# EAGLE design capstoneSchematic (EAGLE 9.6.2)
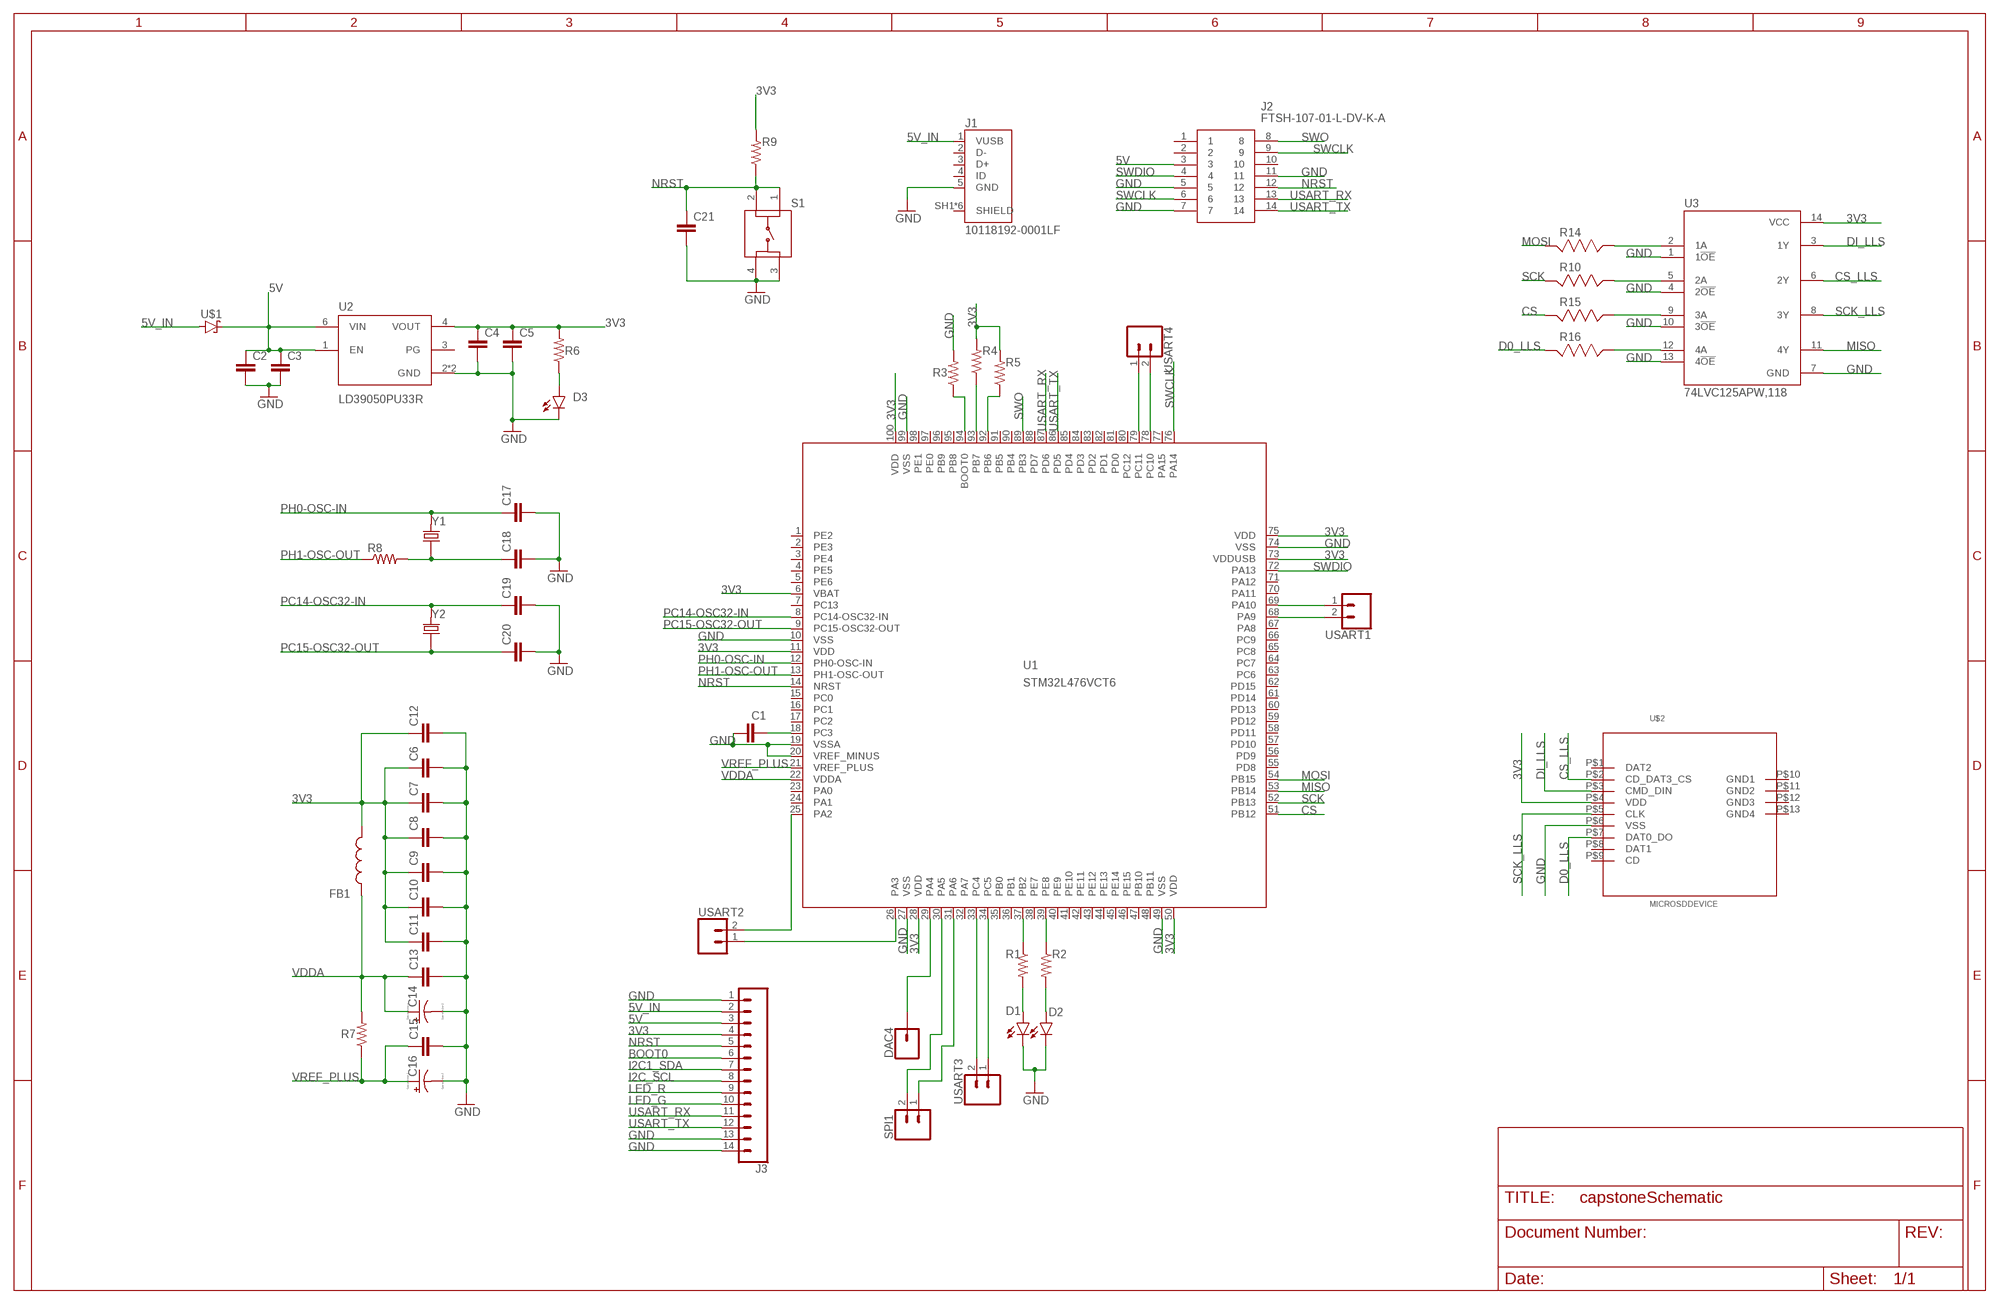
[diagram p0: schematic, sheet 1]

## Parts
C1  CC0603KRX5R7BB105  [CAPC1608X90]
C2  CC0603KRX5R7BB105  [CAPC1608X90]
C3  CC0402KRX7R7BB104  [CAPC1005X55N]
C4  CC0603KRX5R7BB105  [CAPC1608X90]
C5  CC0402KRX7R7BB104  [CAPC1005X55N]
C6  CC0402KRX7R7BB104  [CAPC1005X55N]
C7  CC0402KRX7R7BB104  [CAPC1005X55N]
C8  CC0402KRX7R7BB104  [CAPC1005X55N]
C9  CC0402KRX7R7BB104  [CAPC1005X55N]
C10  CC0402KRX7R7BB104  [CAPC1005X55N]
C11  CC0402KRX7R7BB104  [CAPC1005X55N]
C12  CC0603KRX5R7BB105  [CAPC1608X90]
C13  CC0402KRX7R7BB104  [CAPC1005X55N]
C14  TAJA105K016RNJ  [CAPPM3216X180N]
C15  CC0402KRX7R7BB104  [CAPC1005X55N]
C16  TAJA105K016RNJ  [CAPPM3216X180N]
C17  CC0402JRNPO9BN200  [CAPC1005X55N]
C18  CC0402JRNPO9BN200  [CAPC1005X55N]
C19  CC0402CRNPO9BN4R7  [CAPC1005X55N]
C20  CC0402CRNPO9BN4R7  [CAPC1005X55N]
C21  CC0402KRX7R7BB104  [CAPC1005X55N]
D1  SML-P12MTT86  [LED_SML-P11UTT86R]
D2  SML-P12MTT86  [LED_SML-P11UTT86R]
D3  SML-P12MTT86  [LED_SML-P11UTT86R]
DAC4  CONN_01  [1X01]
FB1  BK1608HS601-T  [BEADC1608X95N]
J1  10118192-0001LF  [AMPHENOL_10118192-0001LF]
J2  FTSH-107-01-L-DV-K-A  [FTSH10701LDVKA]
J3  CONN_14  [1X14]
R1  RC0402FR-071KL  [RESC1005X40N]
R2  RC0402FR-071KL  [RESC1005X40N]
R3  RC0402FR-071KL  [RESC1005X40N]
R4  RC0402FR-071KL  [RESC1005X40N]
R5  RC0402FR-071KL  [RESC1005X40N]
R6  RC0402FR-071KL  [RESC1005X40N]
R7  RC0402FR-071KL  [RESC1005X40N]
R8  RC0402FR-072KL  [RESC1005X40N]
R9  RC0402FR-0710KL  [RESC1005X40N]
R10  RC0402FR-073K3L  [RESC1005X40]
R14  RC0402FR-073K3L  [RESC1005X40]
R15  RC0402FR-073K3L  [RESC1005X40]
R16  RC0402FR-073K3L  [RESC1005X40]
S1  LL3301FF065QJ  [LL3301FF065QJ]
SPI1  CONN_02  [1X02]
U1  STM32L476VCT6  [LQFP100_14X14]
U2  LD39050PU33R  [SON95P300X300X100-7N]
U3  74LVC125APW,118  [IC_74LVC125APW,118]
U$1  STPS1L30A  [DIOM5226X223N]
U$2  MICROSDDEVICE  [MICROSD]
USART1  CONN_02  [1X02]
USART2  CONN_02  [1X02]
USART3  CONN_02  [1X02]
USART4  CONN_02  [1X02]
Y1  ABLS-8.000MHZ-B2-T  [XTAL_ABLS-8.000MHZ-B2-T]
Y2  ECS-.327-12.5-12QS-TR  [XTAL_ECS-.327-12.5-12QS-TR]

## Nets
3V3: C4.1 C5.1 C6.1 C7.1 C8.1 C9.1 C10.1 C11.1 C12.1 FB1.2 J3.4 R4.2 R5.2 R6.2 R9.2 U1.6(VBAT) U1.11(VDD) U1.28(VDD) U1.50(VDD) U1.73(VDDUSB) U1.75(VDD) U1.100(VDD) U2.4(VOUT) U3.14(VCC) U$2.P$4(VDD)
5V: C2.1 C3.1 J2.3 J3.3 U2.1(EN) U2.6(VIN) U$1.1(C)
5V_IN: J1.1(VUSB) J3.2 U$1.2(A)
BOOT0: J3.6
CS: R15.1 U1.51(PB12)
CS_LLS: U3.6(2Y) U$2.P$2(CD_DAT3_CS)
D0_LLS: R16.1 U$2.P$7(DAT0_DO)
DI_LLS: U3.3(1Y) U$2.P$3(CMD_DIN)
GND: C1.1 C2.2 C3.2 C4.2 C5.2 C6.2 C7.2 C8.2 C9.2 C10.2 C11.2 C12.2 C13.2 C14.C(-) C15.2 C16.C(-) C17.2 C18.2 C19.2 C20.2 C21.2 D1.C D2.C D3.C J1.5(GND) J2.5 J2.7 J2.11 J3.1 J3.13 J3.14 R3.2 S1.3 S1.4 U1.10(VSS) U1.19(VSSA) U1.20(VREF_MINUS) U1.27(VSS) U1.49(VSS) U1.74(VSS) U1.99(VSS) U2.2(GND) U2.7(GND) U3.1(1!OE) U3.4(2!OE) U3.7(GND) U3.10(3!OE) U3.13(4!OE) U$2.P$6(VSS)
I2C1_SDA: J3.7
I2C_SCL: J3.8
LED_G: J3.10
LED_R: J3.9
MISO: U1.53(PB14) U3.11(4Y)
MOSI: R14.1 U1.54(PB15)
N$1: R2.1 U1.39(PE8)
N$2: R1.1 U1.37(PB2)
N$3: D1.A R1.2
N$4: D2.A R2.2
N$5: R3.1 U1.94(BOOT0)
N$6: R4.1 U1.93(PB7)
N$7: R5.1 U1.92(PB6)
N$8: D3.A R6.1
N$9: U1.33(PC4) USART3.2
N$10: C1.2 U1.18(PC3)
N$11: U1.34(PC5) USART3.1
N$12: C18.1 R8.2 Y1.1
N$13: R14.2 U3.2(1A)
N$14: U1.78(PC10) USART4.2
N$15: DAC4.1 U1.29(PA4)
N$16: U1.79(PC11) USART4.1
N$17: SPI1.2 U1.30(PA5)
N$18: SPI1.1 U1.31(PA6)
N$19: U1.69(PA10) USART1.1
N$20: U1.68(PA9) USART1.2
N$22: U1.25(PA2) USART2.2
N$23: U1.26(PA3) USART2.1
N$24: R10.2 U3.5(2A)
N$25: R15.2 U3.9(3A)
N$26: R16.2 U3.12(4A)
NRST: C21.1 J2.12 J3.5 R9.1 S1.1 S1.2 U1.14(NRST)
PC14-OSC32-IN: C19.1 U1.8(PC14-OSC32-IN) Y2.2
PC15-OSC32-OUT: C20.1 U1.9(PC15-OSC32-OUT) Y2.1
PH0-OSC-IN: C17.1 U1.12(PH0-OSC-IN) Y1.2
PH1-OSC-OUT: R8.1 U1.13(PH1-OSC-OUT)
SCK: R10.1 U1.52(PB13)
SCK_LLS: U3.8(3Y) U$2.P$5(CLK)
SWCLK: J2.6 J2.9 U1.76(PA14)
SWDIO: J2.4 U1.72(PA13)
SWO: J2.8 U1.89(PB3)
USART_RX: J2.13 J3.11 U1.87(PD6)
USART_TX: J2.14 J3.12 U1.86(PD5)
VDDA: C13.1 C14.A(+) FB1.1 R7.2 U1.22(VDDA)
VREF_PLUS: C15.1 C16.A(+) R7.1 U1.21(VREF_PLUS)
Unconnected: J1.2(D-) J1.3(D+) J1.4(ID) J1.SH1(SHIELD) J1.SH2(SHIELD) J1.SH3(SHIELD) J1.SH4(SHIELD) J1.SH5(SHIELD) J1.SH6(SHIELD) J2.1 J2.2 J2.10 U1.1(PE2) U1.2(PE3) U1.3(PE4) U1.4(PE5) U1.5(PE6) U1.7(PC13) U1.15(PC0) U1.16(PC1) U1.17(PC2) U1.23(PA0) U1.24(PA1) U1.32(PA7) U1.35(PB0) U1.36(PB1) U1.38(PE7) U1.40(PE9) U1.41(PE10) U1.42(PE11) U1.43(PE12) U1.44(PE13) U1.45(PE14) U1.46(PE15) U1.47(PB10) U1.48(PB11) U1.55(PD8) U1.56(PD9) U1.57(PD10) U1.58(PD11) U1.59(PD12) U1.60(PD13) U1.61(PD14) U1.62(PD15) U1.63(PC6) U1.64(PC7) U1.65(PC8) U1.66(PC9) U1.67(PA8) U1.70(PA11) U1.71(PA12) U1.77(PA15) U1.80(PC12) U1.81(PD0) U1.82(PD1) U1.83(PD2) U1.84(PD3) U1.85(PD4) U1.88(PD7) U1.90(PB4) U1.91(PB5) U1.95(PB8) U1.96(PB9) U1.97(PE0) U1.98(PE1) U2.3(PG) U$2.P$1(DAT2) U$2.P$8(DAT1) U$2.P$9(CD) U$2.P$10(GND1) U$2.P$11(GND2) U$2.P$12(GND3) U$2.P$13(GND4)

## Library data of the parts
C1 C2 C4 C12 = ce-capstone:CC0603KRX5R7BB105: CAPACITOR CERAMIC, 1µF, 10V, X5R, 0603; Dielectric Characteristic:X5R; Capacitance:1µF; Capacitance Tolerance:± 10%; Voltage Rating:16V; Temperature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; DESCRIPTION: 1µF ±10% 16V Ceramic Capacitor X5R 0603 _1608 Metric_; DIGI-KEY_PART_NUMBER: 311-1444-1-ND; DIGI-KEY_PURCHASE_URL: https://www.digikey.com/product-detail/en/yageo/CC0603KRX5R7BB105/311-1444-1-ND/2833750?utm_source=snapeda&utm_medium=aggregator&utm_campaign=symbol; MF: Yageo; MP: CC0603KRX5R7BB105; PACKAGE: 0603 Yageo
C3 C5-C11 C13 C15 C21 = ce-capstone:CC0402KRX7R7BB104: .1UF 16V 10% 0402; DESCRIPTION: 0.1µF ±10% 16V Ceramic Capacitor X7R 0402 _1005 Metric_; DIGI-KEY_PART_NUMBER: 311-1338-1-ND; DIGI-KEY_PURCHASE_URL: https://www.digikey.com/product-detail/en/yageo/CC0402KRX7R7BB104/311-1338-1-ND/2103122?utm_source=snapeda&utm_medium=aggregator&utm_campaign=symbol; MF: Yageo; MP: CC0402KRX7R7BB104; PACKAGE: 0402 Yageo
C14 C16 = ce-capstone:TAJA105K016RNJ: Capacitor tantalum TAJ 1206 1uF 16V AVX 1uF SMD Solid MnO2 Tantalum Electrolytic Capacitor, 16 V dc +/-10%, TAJ Series; ALLIED_NUMBER: 70474975; ALLIED_PRICE-STOCK: https://www.alliedelec.com/avx-taja105k016r/70474975/; DESCRIPTION: Capacitor tantalum TAJ 1206 1uF 16V AVX 1uF SMD Solid MnO2 Tantalum Electrolytic Capacitor, 16 V dc +/-10%, TAJ Series; HEIGHT: 1.8mm; MANUFACTURER_NAME: AVX; MANUFACTURER_PART_NUMBER: TAJA105K016RNJ; MOUSER_PART_NUMBER: 581-TAJA105K016RNJ; MOUSER_PRICE-STOCK: https://www.mouser.com/Search/Refine.aspx?Keyword=581-TAJA105K016R; RS_PART_NUMBER: 6992804P; RS_PRICE-STOCK: http://uk.rs-online.com/web/p/products/6992804P
C17 C18 = ce-capstone:CC0402JRNPO9BN200: CAPACITOR CERAMIC 20PF 50V, C0G, 0402; Dielectric Characteristic:C0G / NP0; Capacitance:20pF; Capacitance Tolerance:± 5%; Voltage Rating:50V; Capacitor Case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; DESCRIPTION: 20pF ±5% 50V Ceramic Capacitor C0G, NP0 0402 _1005 Metric_; DIGI-KEY_PART_NUMBER: 311-1417-1-ND; DIGI-KEY_PURCHASE_URL: https://www.digikey.com/product-detail/en/yageo/CC0402JRNPO9BN200/311-1417-1-ND/2833723?utm_source=snapeda&utm_medium=aggregator&utm_campaign=symbol; MF: Yageo; MP: CC0402JRNPO9BN200; PACKAGE: 0402 Yageo
C19 C20 = ce-capstone:CC0402CRNPO9BN4R7: 0402 4.7 pF 50 V ±0.25 pF Tolerance NP0 SMT Multilayer Ceramic Capacitor; DESCRIPTION: 4.7pF ±0.25pF 50V Ceramic Capacitor C0G, NP0 0402 _1005 Metric_; DIGI-KEY_PART_NUMBER: 311-1367-1-ND; DIGI-KEY_PURCHASE_URL: https://www.digikey.com/product-detail/en/yageo/CC0402CRNPO9BN4R7/311-1367-1-ND/2103151?utm_source=snapeda&utm_medium=aggregator&utm_campaign=symbol; MF: Yageo; MP: CC0402CRNPO9BN4R7; PACKAGE: 0402 Yageo
D1-D3 = ce-capstone:SML-P12MTT86: SML-P1 Series Red 0402 Clear 60 mcd 2 V Surface Mount PICOLED LED; AVAILABILITY: Unavailable; DESCRIPTION: Green 572nm LED Indication - Discrete 2V 0402 _1006 Metric_; MF: Rohm; MP: SML-P12MTT86; PACKAGE: 0402 Rohm; PRICE: None
DAC4 = SparkFun-Connectors:CONN_01: Single connection point. Often used as Generic Header-pin footprint for 0.1 inch spaced/style header connections
FB1 = ce-capstone:BK1608HS601-T: Ferrite Chip Bead(Lead Free); DESCRIPTION: Ferrite Chip Bead(Lead Free); HEIGHT: 0.95mm; MANUFACTURER_NAME: Taiyo Yuden; MANUFACTURER_PART_NUMBER: BK1608HS601-T
J1 = ce-capstone:10118192-0001LF: Single Port 5 Contact Horizontal Right Angle Shielded Micro B USB 2.0 Connector; AVAILABILITY: Unavailable; DESCRIPTION: USB - micro B USB 2.0 Receptacle Connector 5 Position Surface Mount, Right Angle; MF: Amphenol ICC; MP: 10118192-0001LF; PACKAGE: None; PRICE: None
J2 = ce-capstone:FTSH-107-01-L-DV-K-A: Headers & Wire Housings .050" Micro Terminal Strip Source: Datasheet; DESCRIPTION: Headers & Wire Housings .050" Micro Terminal Strip; HEIGHT: 5.97mm; MANUFACTURER_NAME: SAMTEC; MANUFACTURER_PART_NUMBER: FTSH-107-01-L-DV-K-A; MOUSER_PART_NUMBER: 200-FTSH10701LDVKA; MOUSER_PRICE-STOCK: https://www.mouser.com/Search/Refine.aspx?Keyword=200-FTSH10701LDVKA
J3 = SparkFun-Connectors:CONN_14: Multi connection point. Often used as Generic Header-pin footprint for 0.1 inch spaced/style header connections On any of the 0.1 inch spaced packages, you can populate with these: Break Away Headers - Straight (PRT-00116) Break Away Male Headers - Right Angle (PRT-00553) Female Headers (PRT-00115)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
R1-R7 = ce-capstone:RC0402FR-071KL: RES SMD 1k OHM 1% 1/16W 0402; DESCRIPTION: 510 Ohms ±1% 0.063W, 1/16W Chip Resistor 0402 _1005 Metric_ Moisture Resistant Thick Film; DIGI-KEY_PART_NUMBER: 311-510LRCT-ND; DIGI-KEY_PURCHASE_URL: https://www.digikey.com/product-detail/en/yageo/RC0402FR-07510RL/311-510LRCT-ND/729579?utm_source=snapeda&utm_medium=aggregator&utm_campaign=symbol; MF: Yageo; MP: RC0402FR-07510RL; PACKAGE: 1005 Panasonic Electronic Components
R8 = ce-capstone:RC0402FR-072KL: RES SMD 2k OHM 1% 1/16W 0402; DESCRIPTION: 510 Ohms ±1% 0.063W, 1/16W Chip Resistor 0402 _1005 Metric_ Moisture Resistant Thick Film; DIGI-KEY_PART_NUMBER: 311-510LRCT-ND; DIGI-KEY_PURCHASE_URL: https://www.digikey.com/product-detail/en/yageo/RC0402FR-07510RL/311-510LRCT-ND/729579?utm_source=snapeda&utm_medium=aggregator&utm_campaign=symbol; MF: Yageo; MP: RC0402FR-07510RL; PACKAGE: 1005 Panasonic Electronic Components
R9 = ce-capstone:RC0402FR-0710KL: RES SMD 10k OHM 1% 1/16W 0402; DESCRIPTION: 510 Ohms ±1% 0.063W, 1/16W Chip Resistor 0402 _1005 Metric_ Moisture Resistant Thick Film; DIGI-KEY_PART_NUMBER: 311-510LRCT-ND; DIGI-KEY_PURCHASE_URL: https://www.digikey.com/product-detail/en/yageo/RC0402FR-07510RL/311-510LRCT-ND/729579?utm_source=snapeda&utm_medium=aggregator&utm_campaign=symbol; MF: Yageo; MP: RC0402FR-07510RL; PACKAGE: 1005 Panasonic Electronic Components
R10 R14-R16 = RC0402FR-073K3L:RC0402FR-073K3L: RC Series 0402 0.063 W 3.3 kOhms ±1% ±100 ppm/°C SMT Thick Film Chip Resistor; MANUFACTURER: YAGEO
S1 = ce-capstone:LL3301FF065QJ: Pushbutton Switches 50mA 12VDC F065 7.0mm J-Lead Source: Datasheet; DESCRIPTION: Pushbutton Switches 50mA 12VDC F065 7.0mm J-Lead; HEIGHT: 7.3mm; MANUFACTURER_NAME: E-Switch; MANUFACTURER_PART_NUMBER: LL3301FF065QJ; MOUSER_PART_NUMBER: 612-LL3301FF065QJ; MOUSER_PRICE-STOCK: https://www.mouser.com/Search/Refine.aspx?Keyword=612-LL3301FF065QJ
SPI1 USART1-USART4 = SparkFun-Connectors:CONN_02: Multi connection point. Often used as Generic Header-pin footprint for 0.1 inch spaced/style header connections
U1 = ce-capstone:STM32L476V*: STM32L476VX LQFP100 Datasheet STM32L476XX; FARNELL: 2518171; FLASH: 256kB; SRAM: 128kB
U2 = ce-capstone:LD39050PU33R: LD39050 Series 500 mA 3.3 V Fixed Low Noise LDO Voltage Regulator - DFN-6; AVAILABILITY: Unavailable; DESCRIPTION: Linear Voltage Regulator IC 1 Output 500mA 6-DFN _3x3_; MF: STMicroelectronics; MP: LD39050PU33R; PACKAGE: DFN-6 STMicroelectronics; PRICE: None
U3 = 74LVC125APW_118:74LVC125APW,118: Check availability Check availability Check availability; AVAILABILITY: In Stock; CHECK_PRICES: https://www.snapeda.com/parts/74LVC125APW,118/Nexperia/view-part/?ref=eda; DESCRIPTION: Buffer, Non-Inverting 4 Element 1 Bit per Element 3-State Output 14-TSSOP; MF: Nexperia USA Inc.; MP: 74LVC125APW,118; PACKAGE: TSSOP14-14 Nexperia USA Inc.; PRICE: None; PURCHASE-URL: https://www.snapeda.com/api/url_track_click_mouser/?unipart_id=5248541&manufacturer=Nexperia USA Inc.&part_name=74LVC125APW,118&search_term=None; SNAPEDA_LINK: https://www.snapeda.com/parts/74LVC125APW,118/Nexperia/view-part/?ref=snap
U$1 = ce-capstone:STPS1L30A
U$2 = MicroSDFootprint:MICROSDDEVICE
Y1 = ce-capstone:ABLS-8.000MHZ-B2-T: Crystal 8MHz Â±20ppm (Tol) Â±50ppm (Stability) 18pF FUND 80Ohm 2-Pin HC-49/US SMD T/R; AVAILABILITY: Unavailable; DESCRIPTION: 8MHz ±20ppm Crystal 18pF 80 Ohms HC-49/US; MF: Abracon LLC; MP: ABLS-8.000MHZ-B2; PACKAGE: HC-49/US Abracon LLC; PRICE: None
Y2 = ce-capstone:ECS-.327-12.5-12QS-TR: SMD CRYSTAL 32.768 KHz; AVAILABILITY: Unavailable; DESCRIPTION: 32.768kHz ±20ppm Crystal 12.5pF 90 kOhms 2-SMD, No Lead; MF: ECS Inc.; MP: ECS-.327-12.5-12QS-TR; PACKAGE: SMD-2 ECS International; PRICE: None

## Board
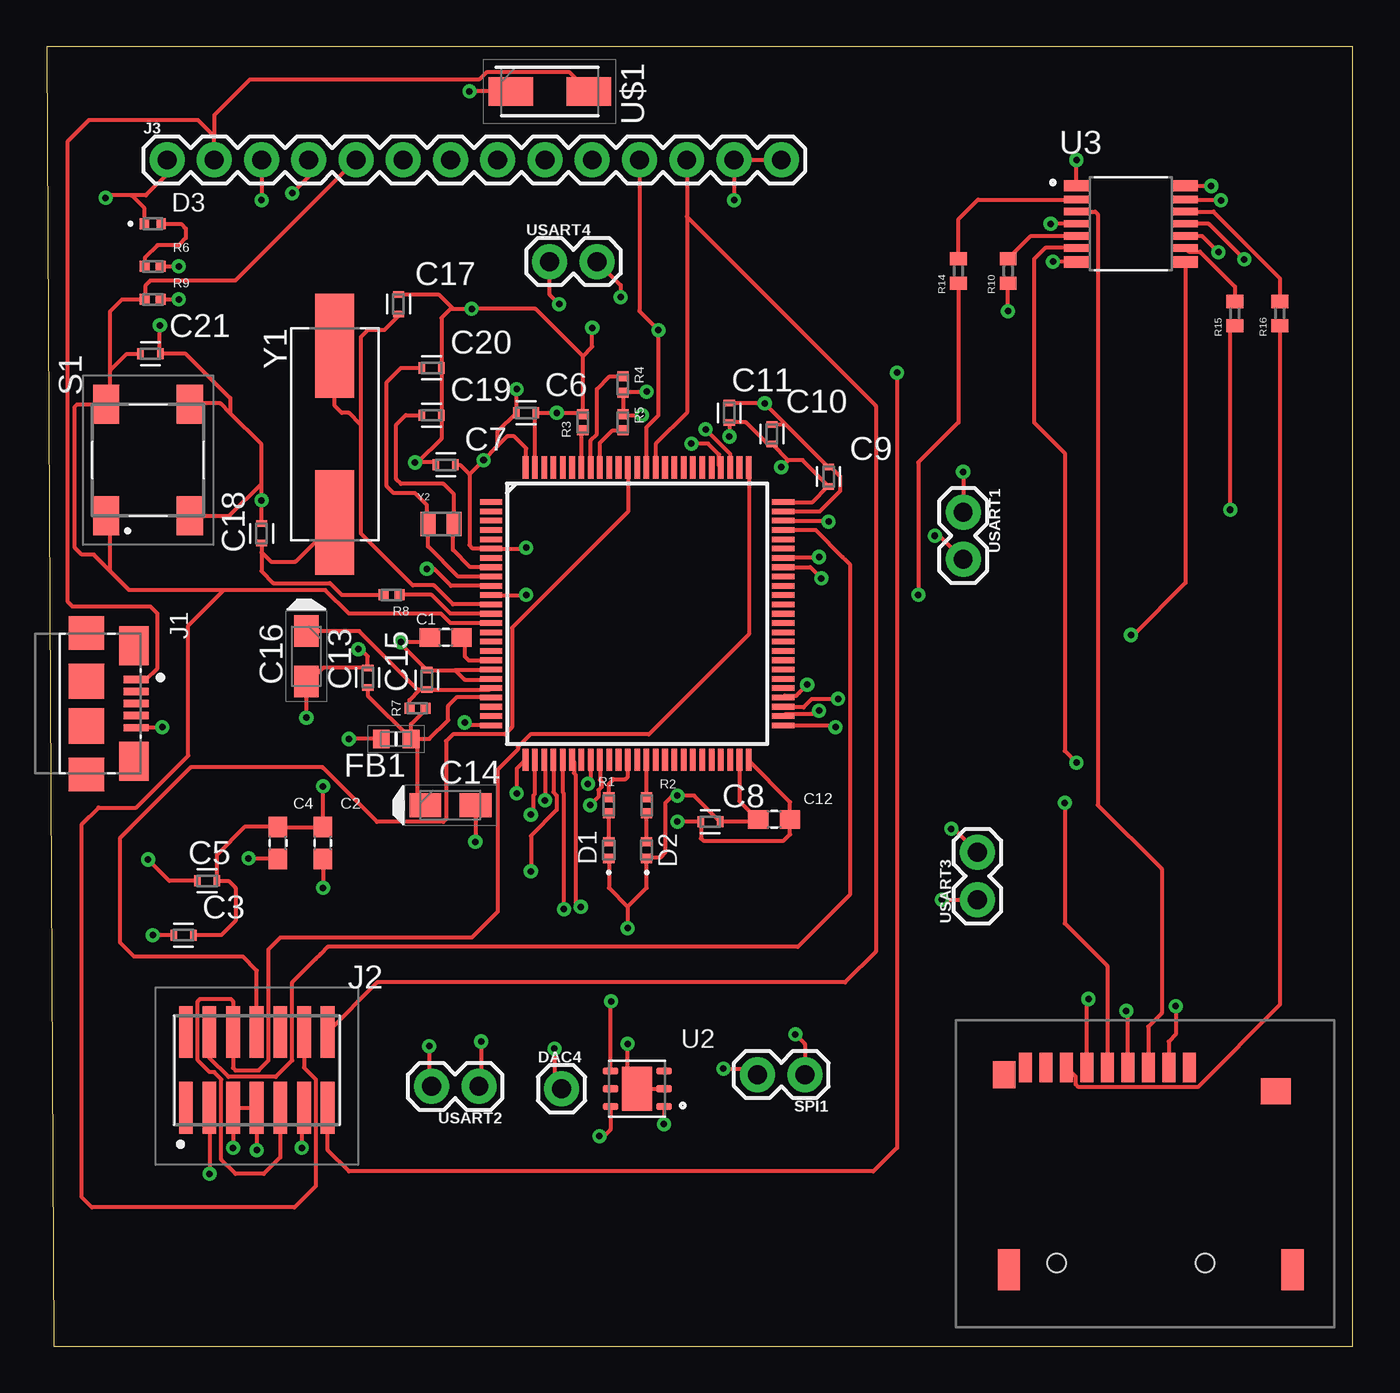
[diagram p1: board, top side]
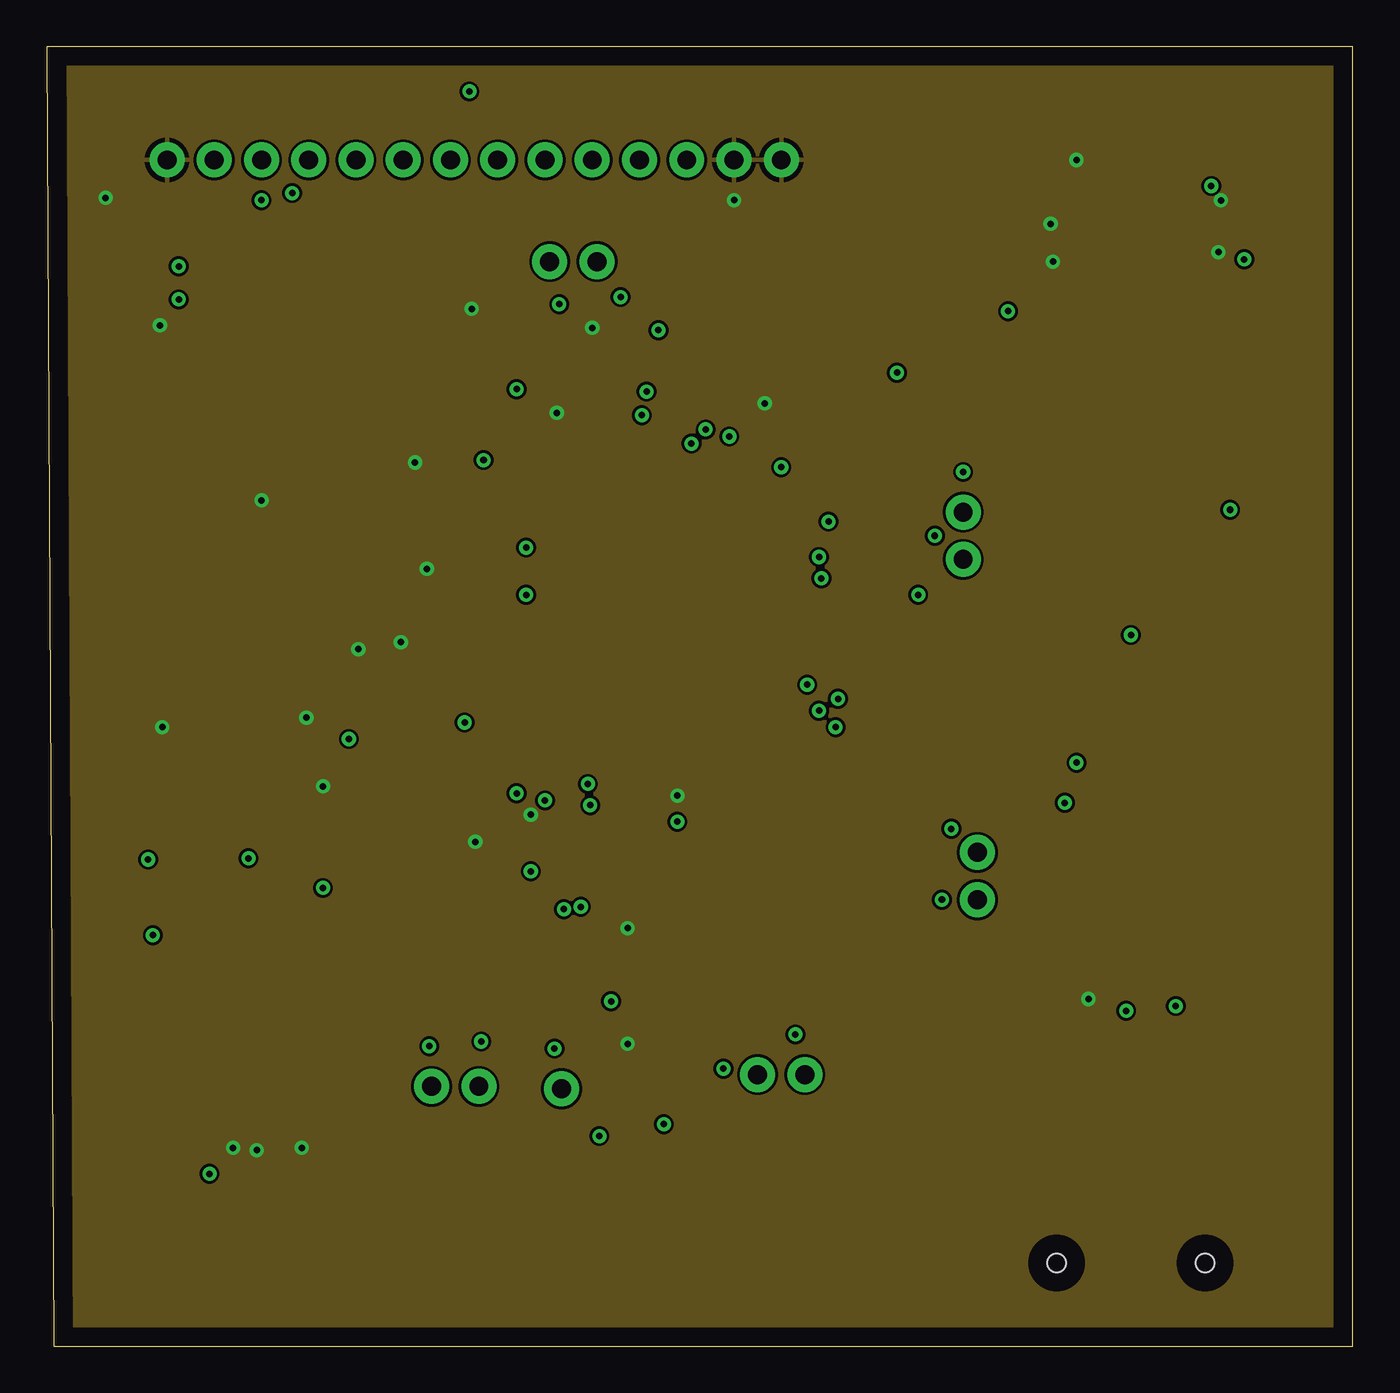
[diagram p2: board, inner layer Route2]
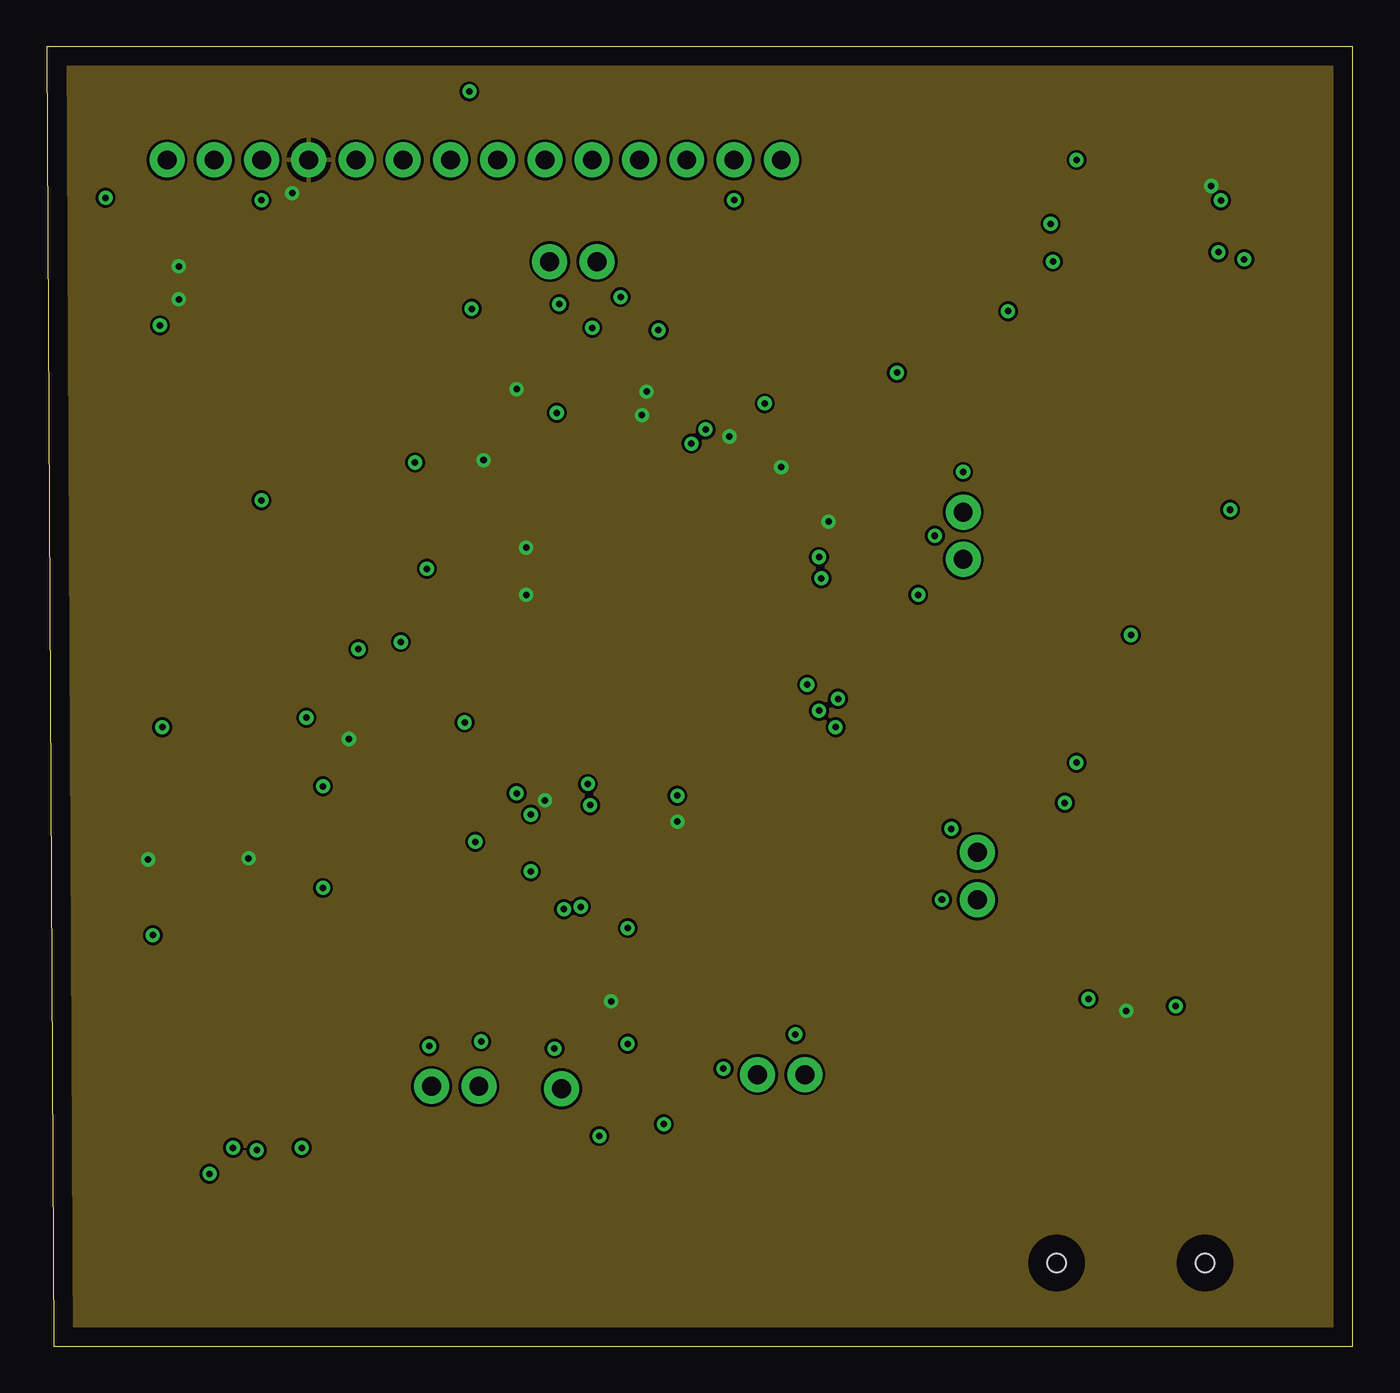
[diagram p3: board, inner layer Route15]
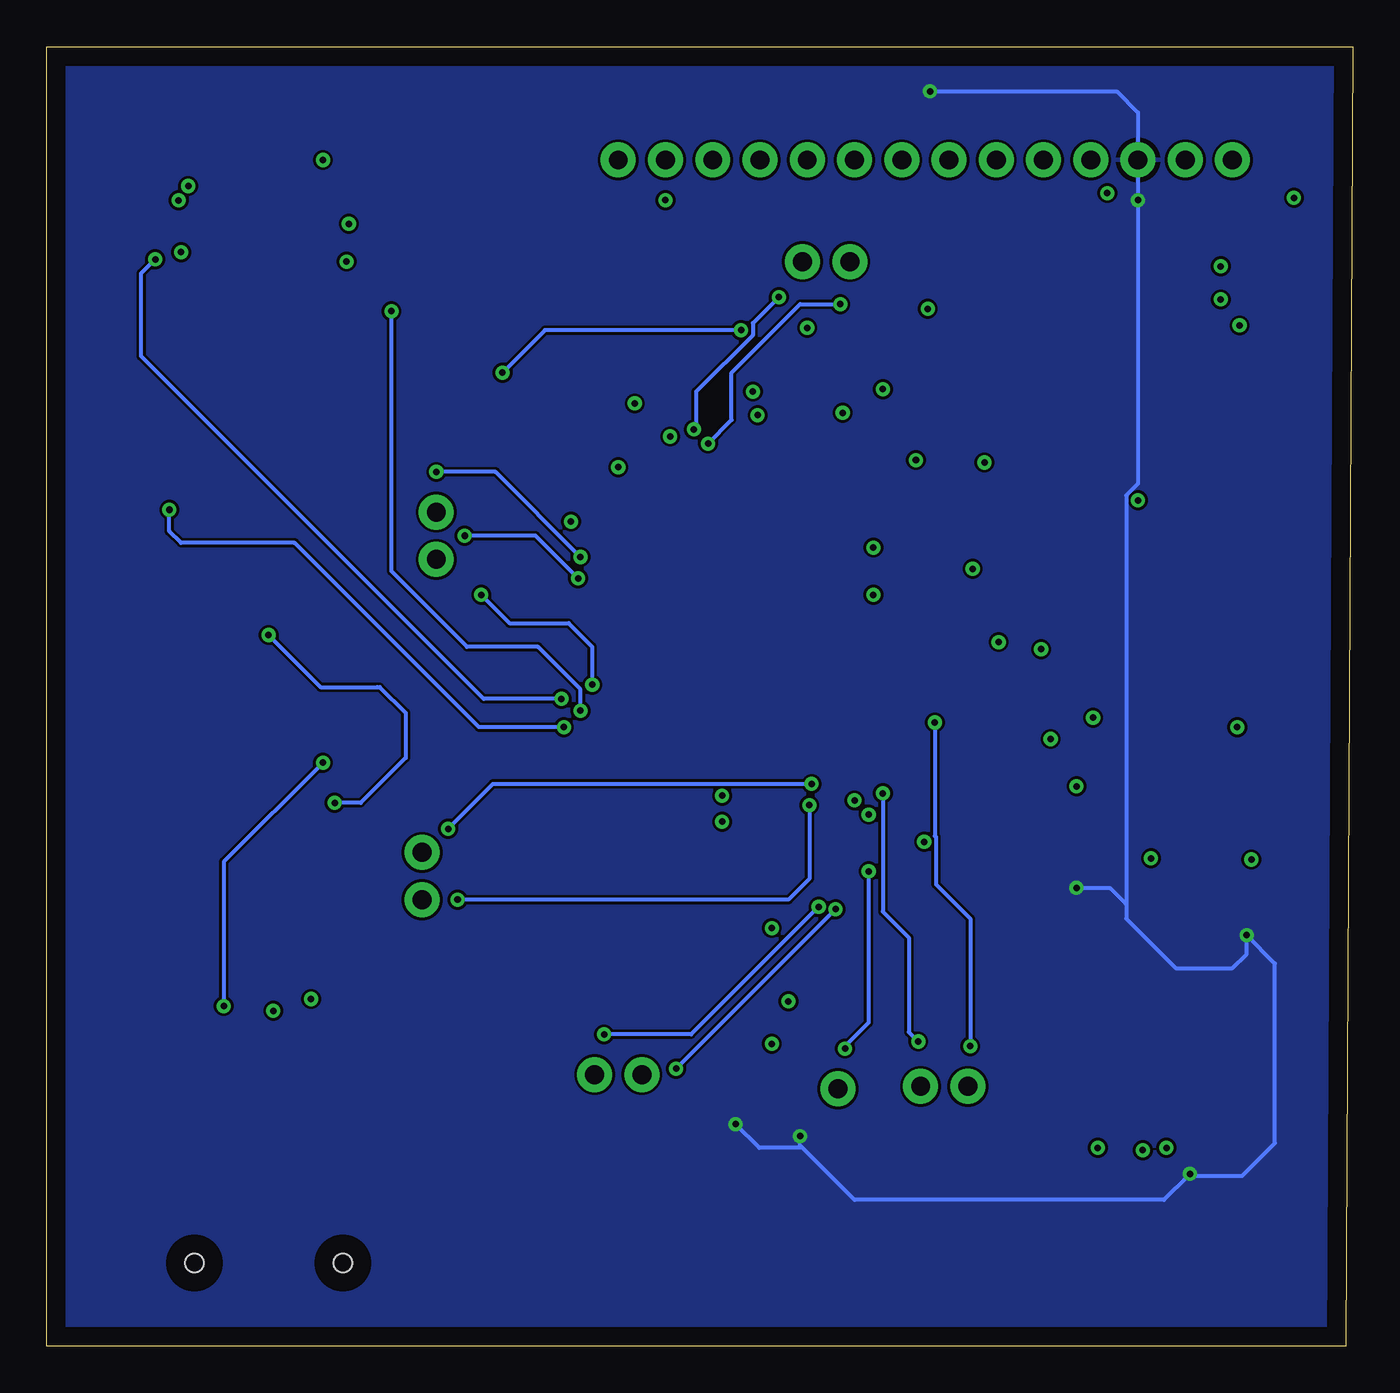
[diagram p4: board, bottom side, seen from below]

Size 70.23 x 69.85 mm. Coordinates in mm from the lower left corner, seen from the top.
Outline: 0.38,0 70.23,0 70.23,69.85 0,69.85 0.38,0
Copper layers (1+2*15+16): Top 0.035mm / dielectric 1.5mm / Route2 0.035mm / dielectric 0.15mm / Route15 0.035mm / dielectric 0.2mm / Bottom 0.035mm
Design rules "default *": minimum track width 8mil, minimum drill 0.35mm, track to track 6mil, track to pad 6mil, pad to pad 6mil, via to via 6mil, smd to smd 6mil, copper to edge 40mil, drill to drill 6mil, minimum pad ring 10mil, minimum via ring 8mil, stop-mask expansion 4mil, vias tented up to drill 0mil, thermal gap 10mil

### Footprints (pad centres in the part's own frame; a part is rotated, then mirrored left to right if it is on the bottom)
CAPC1608X90 = smd 1.1 x 1: 1 -0.85,0; 2 0.85,0
CAPC1005X55N = smd 0.35 x 0.6: 1 -0.525,0; 2 0.525,0
CAPPM3216X180N = smd 1.7 x 1.3: A -1.35,0; C 1.35,0
LED_SML-P11UTT86R = smd 0.5 x 0.6: A 0.45,0; C -0.45,0
1X01 = drill 1.016 pad 1.88: 1 0,0
BEADC1608X95N = smd 0.9 x 1: 1 -0.8,0; 2 0.8,0
AMPHENOL_10118192-0001LF = smd 0.4 x 1.35: 1 -1.3,0; 2 -0.65,0; 3 0,0; 4 0.65,0; 5 1.3,0 | smd 2.1 x 1.6: SH1 -3.1,-0.125; SH2 3.1,-0.125 | smd 1.8 x 1.9: SH3 -3.8,-2.675; SH6 3.8,-2.675 | smd 1.9 x 1.9: SH4 -1.2,-2.675; SH5 1.2,-2.675
FTSH10701LDVKA = smd 0.74 x 2.79: 1 -3.81,-2.035; 2 -3.81,2.035; 3 -2.54,-2.035; 4 -2.54,2.035; 5 -1.27,-2.035; 6 -1.27,2.035; 7 0,-2.035; 8 0,2.035; 9 1.27,-2.035; 10 1.27,2.035; 11 2.54,-2.035; 12 2.54,2.035; 13 3.81,-2.035; 14 3.81,2.035
1X14 = drill 1.016 pad 1.88: 1 0,0; 2 2.54,0; 3 5.08,0; 4 7.62,0; 5 10.16,0; 6 12.7,0; 7 15.24,0; 8 17.78,0; 9 20.32,0; 10 22.86,0; 11 25.4,0; 12 27.94,0; 13 30.48,0; 14 33.02,0
RESC1005X40N = smd 0.54 x 0.6: 1 -0.432,0; 2 0.432,0
RESC1005X40 = smd 0.7 x 0.9: 1 -0.65,0; 2 0.65,0
LL3301FF065QJ = smd 2.1 x 1.4: 1 -3,2.25; 2 3,2.25; 3 -3,-2.25; 4 3,-2.25
1X02 = drill 1.016 pad 1.88: 1 0,0; 2 2.54,0
LQFP100_14X14 = smd 1.2 x 0.3: 1 -7.85,6; 2 -7.85,5.5; 3 -7.85,5; 4 -7.85,4.5; 5 -7.85,4; 6 -7.85,3.5; 7 -7.85,3; 8 -7.85,2.5; 9 -7.85,2; 10 -7.85,1.5; 11 -7.85,1; 12 -7.85,0.5; 13 -7.85,0; 14 -7.85,-0.5; 15 -7.85,-1; 16 -7.85,-1.5; 17 -7.85,-2; 18 -7.85,-2.5; 19 -7.85,-3; 20 -7.85,-3.5; 21 -7.85,-4; 22 -7.85,-4.5; 23 -7.85,-5; 24 -7.85,-5.5; 25 -7.85,-6; 51 7.85,-6; 52 7.85,-5.5; 53 7.85,-5; 54 7.85,-4.5; 55 7.85,-4; 56 7.85,-3.5; 57 7.85,-3; 58 7.85,-2.5; 59 7.85,-2; 60 7.85,-1.5; 61 7.85,-1; 62 7.85,-0.5; 63 7.85,0; 64 7.85,0.5; 65 7.85,1; 66 7.85,1.5; 67 7.85,2; 68 7.85,2.5; 69 7.85,3; 70 7.85,3.5; 71 7.85,4; 72 7.85,4.5; 73 7.85,5; 74 7.85,5.5; 75 7.85,6 | smd 0.3 x 1.2: 26 -6,-7.85; 27 -5.5,-7.85; 28 -5,-7.85; 29 -4.5,-7.85; 30 -4,-7.85; 31 -3.5,-7.85; 32 -3,-7.85; 33 -2.5,-7.85; 34 -2,-7.85; 35 -1.5,-7.85; 36 -1,-7.85; 37 -0.5,-7.85; 38 0,-7.85; 39 0.5,-7.85; 40 1,-7.85; 41 1.5,-7.85; 42 2,-7.85; 43 2.5,-7.85; 44 3,-7.85; 45 3.5,-7.85; 46 4,-7.85; 47 4.5,-7.85; 48 5,-7.85; 49 5.5,-7.85; 50 6,-7.85; 76 6,7.85; 77 5.5,7.85; 78 5,7.85; 79 4.5,7.85; 80 4,7.85; 81 3.5,7.85; 82 3,7.85; 83 2.5,7.85; 84 2,7.85; 85 1.5,7.85; 86 1,7.85; 87 0.5,7.85; 88 0,7.85; 89 -0.5,7.85; 90 -1,7.85; 91 -1.5,7.85; 92 -2,7.85; 93 -2.5,7.85; 94 -3,7.85; 95 -3.5,7.85; 96 -4,7.85; 97 -4.5,7.85; 98 -5,7.85; 99 -5.5,7.85; 100 -6,7.85
SON95P300X300X100-7N = smd 0.84 x 0.4: 1 -1.435,0.95; 2 -1.435,0; 3 -1.435,-0.95; 4 1.435,-0.95; 5 1.435,0; 6 1.435,0.95 | smd 1.625 x 2.365: 7 0,0
IC_74LVC125APW,118 = smd 1.35 x 0.6: 1 -2.925,2.05; 7 -2.925,-2.05; 8 2.925,-2.05; 14 2.925,2.05 | smd 1.35 x 0.4: 2 -2.925,1.3; 3 -2.925,0.65; 4 -2.925,0; 5 -2.925,-0.65; 6 -2.925,-1.3; 9 2.925,-1.3; 10 2.925,-0.65; 11 2.925,0; 12 2.925,0.65; 13 2.925,1.3
DIOM5226X223N = smd 2.4 x 1.55: 1 -2.1,0; 2 2.1,0
MICROSD = smd 1.6 x 0.7: P$1 -3.81,1.1; P$2 -3.81,0; P$3 -3.81,-1.1; P$4 -3.81,-2.2; P$5 -3.81,-3.3; P$6 -3.81,-4.4; P$7 -3.81,-5.5; P$8 -3.81,-6.6; P$9 -3.81,-7.7 | smd 1.45 x 1.2: P$10 -3.41,-8.85 | smd 1.4 x 1.6: P$11 -2.54,5.75 | smd 2.2 x 1.2: P$12 7.06,6.65; P$13 7.06,-8.59 | hole 1: 6.69,1.95; 6.69,-6.03
XTAL_ABLS-8.000MHZ-B2-T = smd 5.6 x 2.1: 1 -4.75,0; 2 4.75,0
XTAL_ECS-.327-12.5-12QS-TR = smd 0.8 x 1.3: 1 -0.7,0; 2 0.7,0

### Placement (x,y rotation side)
C1  21.46,38.1 0 top
C2  14.86,27.05 90 top
C3  7.37,22.1 0 top
C4  12.45,27.05 90 top
C5  8.64,25.02 0 top
C6  25.78,50.16 0 top
C7  21.46,47.37 180 top
C8  35.69,28.19 0 top
C9  42.04,46.74 90 top
C10  38.99,49.02 90 top
C11  36.7,50.16 90 top
C12  39.12,28.32 180 top
C13  17.27,35.94 90 top
C14  21.72,29.08 0 top
C15  20.45,35.81 90 top
C16  13.97,37.08 270 top
C17  18.92,56.01 90 top
C18  11.56,43.69 90 top
C19  20.7,50.04 0 top
C20  20.7,52.58 0 top
C21  5.59,53.34 0 top
D1  30.23,26.67 90 top
D2  32.26,26.67 90 top
D3  5.71,60.33 0 top
DAC4  27.69,13.84 0 top
FB1  18.8,32.64 180 top
J1  4.83,34.54 270 top
J2  11.3,14.86 0 top
J3  6.48,63.75 0 top
R1  30.23,29.08 270 top
R2  32.26,29.08 270 top
R3  28.83,49.66 90 top
R4  30.99,51.69 270 top
R5  30.99,49.66 90 top
R6  5.71,58.04 0 top
R7  19.94,34.29 0 top
R8  18.54,40.39 180 top
R9  5.71,56.26 0 top
R10  51.69,57.79 90 top
R14  49.02,57.79 90 top
R15  63.88,55.5 90 top
R16  66.29,55.5 90 top
S1  5.46,47.62 90 top
SPI1  40.77,14.61 180 top
U1  31.75,39.37 0 top
U2  31.75,13.84 180 top
U3  58.29,60.33 0 top
U$1  27.05,67.44 0 top
U$2  60.33,11.18 270 top
USART1  49.28,44.83 270 top
USART2  23.24,13.97 180 top
USART3  50.04,24 90 top
USART4  27.05,58.29 0 top
Y1  15.49,49.02 90 top
Y2  21.21,44.2 0 top

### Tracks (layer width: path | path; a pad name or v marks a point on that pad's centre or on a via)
3V3  (via drill 0.35)
  Top 0.203: 22.73,46.86 22.73,43.05 22.92,42.87 U1.6 25.73,42.87 v25.78,42.93 | 22.73,46.86 v23.5,47.62 24.26,48.39 | 24.26,48.39 24.26,49.17 C6.1 25.26,51.42 v25.27,51.44 | U1.50 37.75,31.46 39.97,29.25 C12.1 39.97,27.52 39.62,27.18 35.31,27.18 35.18,27.3 35.18,28.18 C8.1 v33.91,28.19 | U1.75 41.18,45.37 42.02,46.21 C9.1 40.64,47.61 40.64,47.62 39.88,47.62 | 39.88,47.62 39.86,47.62 C10.1 38.75,48.5 37.59,49.66 36.72,49.66 C11.1 v36.7,48.9 | 39.88,47.62 v39.5,47.24 | FB1.2 v16.26,32.64 | v32.26,51.31 31.04,51.31 R4.2 R5.2 31.04,50.04 v32,50.04 | C7.1 22.23,47.37 22.73,46.86 | U1.100 25.78,47.25 25.78,48.26 25.15,48.9 24.77,48.9 24.26,48.39 | U1.28 26.8,31.47 v26.8,29.34 | U2.4 30.32,18.5 v30.35,18.54 | C5.1 6.6,25.02 v5.46,26.16 | J3.4 14.1,62.87 v13.21,61.98 | R9.2 v7.11,56.26 | R6.2 v7.11,58.04 | U1.73 41.99,44.37 v42.04,44.32 | U1.11 25.77,40.37 v25.78,40.39 | C4.1 10.88,26.2 v10.86,26.23 | U3.14 62.59,62.38 v62.61,62.36 | U$2.P$4 58.12,17.95 v58.04,18.03
  pour Route15: 0.76,69.34 69.85,69.34 69.85,0.25 0.76,0.25
5V  (via drill 0.35)
  Top 0.203: U2.1 v33.19,11.94 | U2.6 30.32,11.65 29.97,11.3 v29.72,11.3 | J2.3 v8.76,9.27 | J3.3 v11.56,61.59 | C2.1 v14.86,24.64 | C3.1 v5.71,22.1 | U$1.1 v22.73,67.44
  Bottom 0.203: 12.19,23.75 12.19,45.73 11.56,46.36 v11.56,61.59 11.56,66.29 12.7,67.44 v22.73,67.44 | 12.19,23.75 12.19,22.98 9.53,20.32 6.48,20.32 5.71,21.08 v5.71,22.1 4.19,20.57 4.19,10.92 5.97,9.14 8.89,9.14 | v8.76,9.27 8.89,9.14 | 8.89,9.14 10.16,7.87 26.8,7.87 29.59,10.67 | v29.72,11.3 29.72,10.79 29.59,10.67 | v14.86,24.64 13.08,24.64 12.19,23.75 | v33.19,11.94 31.91,10.67 29.59,10.67
  pour Bottom: 1.14,69.34 69.85,69.34 69.85,0.38 0.89,0.38 0.89,69.47 1.14,69.47
5V_IN
  Top 0.203: J3.2 9.02,65.02 | J1.1 5.3,35.84 5.33,35.81 5.97,36.45 5.97,39.37 5.59,39.75 1.4,39.75 1.14,40.01 1.14,64.77 2.29,65.91 8.13,65.91 9.02,65.02 | U$1.2 28.12,68.47 23.65,68.47 23.25,68.07 10.92,68.07 9.02,66.17 9.02,65.02
CS  (via drill 0.35)
  Top 0.203: U1.51 42.32,33.37 v42.42,33.27 | v63.63,44.96 63.63,54.59 R15.1
  Bottom 0.203: v42.42,33.27 46.99,33.27 56.9,43.18 62.99,43.18 63.63,43.82 v63.63,44.96
CS_LLS  (via drill 0.35)
  Top 0.203: U$2.P$2 60.33,16.38 60.71,16.76 v60.71,18.29 | U3.6 53.69,59.02 53.09,58.42 53.09,49.66 54.74,48.01 54.74,32 v55.37,31.37
  Bottom 0.203: v55.37,31.37 60.71,26.03 v60.71,18.29
D0_LLS
  Top 0.203: U$2.P$7 55.32,14.49 55.32,14.08 55.47,13.93 61.88,13.93 66.29,18.35 R16.1
DI_LLS
  Top 0.203: U$2.P$3 59.23,17.19 59.94,17.91 59.94,25.65 56.52,29.08 56.52,60.83 56.37,60.98 U3.3
GND  (via drill 0.35)
  Top 0.203: J1.5 4.86,33.27 v6.22,33.27 | v10.03,10.67 J2.5 J2.7 v11.3,10.54 | U1.20 23.86,35.83 22.48,35.83 21.97,36.34 | U1.19 23.87,36.34 21.97,36.34 | 21.97,36.34 C15.2 19.05,37.74 v19.05,37.85 20.36,37.85 C1.1 | U1.99 26.25,50.11 C6.2 v27.43,50.16 28.75,50.16 R3.2 28.83,53.21 | C12.2 38.14,28.19 37.85,28.19 | 37.85,28.19 C8.2 34.81,29.59 v33.91,29.59 33.66,29.59 33.27,29.21 33.27,26.54 33.02,26.29 32.33,26.29 D2.C 32.26,24.64 31.24,23.62 | U1.74 41.57,44.87 42.67,45.97 42.67,46.74 42.15,47.26 C9.2 42.02,47.26 39.73,49.55 | C10.2 39.73,49.55 | 39.73,49.55 v38.61,50.67 36.72,50.67 C11.2 | C14.C 23.07,27.23 23.11,27.18 v23.05,27.12 | C16.C 13.97,35.56 | 13.97,35.56 v13.97,33.78 | D1.C 30.23,24.64 31.24,23.62 | 31.24,23.62 v31.24,22.48 | C18.2 v11.56,45.47 11.56,46.36 | C17.2 21.07,56.53 21.84,55.75 | 21.84,55.75 v22.86,55.75 26.29,55.75 28.83,53.21 | 21.84,55.75 21.72,55.75 21.23,55.26 C20.2 C19.2 21.23,48.79 19.94,47.5 v19.81,47.5 20.81,47.5 C7.2 | S1.3 9.83,44.62 11.56,46.36 | 11.56,46.36 11.56,48.47 9.88,50.14 | U2.2 U2.7 31.24,14.35 v31.24,16.26 | 28.83,53.21 29.34,53.72 v29.34,54.74 | U1.10 21.74,40.87 20.83,41.78 v20.45,41.78 | U1.49 37.25,29.3 37.85,28.7 37.85,28.19 | J2.11 13.84,11.68 13.72,11.56 v13.72,10.67 | C3.2 9.4,22.1 10.16,22.86 10.16,24.64 9.78,25.02 C5.2 9.16,26.42 10.69,27.94 12.41,27.94 C4.2 C2.2 v14.86,30.1 | J3.1 6.48,62.99 5.33,61.85 4.57,61.85 | 4.57,61.85 3.3,61.85 v3.17,61.72 | v6.1,54.86 6.1,53.36 C21.2 7.49,53.34 9.88,50.95 9.88,50.14 | D3.C 5.26,61.16 4.57,61.85 | J3.14 J3.13 v36.96,61.59 | v26.04,28.58 26.16,28.7 26.16,29.6 26.25,29.68 U1.27 | S1.4 7.71,50.67 9.35,50.67 9.88,50.14
  Top 0.203: 13.97,35.56 14.88,36.47 C13.2 17.27,37.08 16.89,37.46 v16.76,37.46 | U$2.P$6 55.92,18.59 v56.01,18.67 | U3.1 v55.37,63.75 | U3.4 v53.98,60.33 | U3.7 54.12,58.27 v54.1,58.29 | U3.13 63.09,61.62 v63.13,61.59 | U3.10 62.12,59.68 v62.99,58.8
  pour Route2: 0.76,69.34 69.85,69.34 69.85,0.38 0.76,0.38
MISO  (via drill 0.35)
  Top 0.203: U1.53 39.63,34.34 40.69,34.34 41.15,34.8 v42.55,34.8 | v64.39,58.42 62.48,60.33 U3.11
  Bottom 0.203: v42.55,34.8 46.74,34.8 65.15,53.21 65.15,57.66 v64.39,58.42
MOSI  (via drill 0.35)
  Top 0.203: U1.54 39.7,34.97 40.3,34.97 40.45,35.12 v40.89,35.56 | R14.1 49.02,49.66 46.86,47.5 v46.86,40.39
  Bottom 0.203: v46.86,40.39 45.34,38.86 42.16,38.86 40.89,37.59 v40.89,35.56
N$1
  Top 0.203: R2.1 32.25,29.52 U1.39
N$2
  Top 0.203: R1.1 30.23,30.23 30.48,30.48 31.11,30.48 31.25,30.62 U1.37
N$3
  Top 0.203: D1.A R1.2
N$4
  Top 0.203: D2.A R2.2
N$5
  Top 0.203: U1.94 28.75,49.15 R3.1
N$6
  Top 0.203: U1.93 29.25,48.68 29.59,49.02 29.59,51.44 30.28,52.12 R4.1
N$7
  Top 0.203: U1.92 29.75,48.55 30.43,49.23 R5.1
N$8
  Top 0.203: D3.A 7.24,60.33 7.49,60.07 7.49,59.56 7.11,59.18 5.97,59.18 5.28,58.5 R6.1
N$9  (via drill 0.35)
  Top 0.203: U1.33 29.25,30.37 v29.1,30.23 | v48.64,27.81 48.77,27.81 USART3.2
  Bottom 0.203: v29.1,30.23 v29.11,30.22 46.23,30.22 v48.64,27.81
N$10
  Top 0.203: C1.2 22.48,37.93 22.48,37.08 22.69,36.87 U1.18
N$11  (via drill 0.35)
  Top 0.203: U1.34 29.75,30.45 29.84,30.35 29.84,30.06 29.67,29.89 29.67,29.53 v29.23,29.08 | v48.13,24 USART3.1
  Bottom 0.203: v29.23,29.08 29.23,25.13 30.35,24 v48.13,24
N$12
  Top 0.203: C18.1 11.56,42.67 | 11.56,42.67 11.56,41.66 12.19,41.02 15.24,41.02 15.88,40.39 R8.2 | 11.56,42.67 12.06,42.16 13.39,42.16 Y1.1
N$13
  Top 0.203: R14.2 49.02,60.58 50.07,61.62 U3.2
N$14  (via drill 0.35)
  Top 0.203: USART4.2 30.86,57.02 v30.86,56.39 | v35.43,49.28 36.07,48.64 36.07,48.63 36.75,47.95 U1.78
  Bottom 0.203: v30.86,56.39 32.26,54.99 32.26,54.35 35.31,51.3 35.31,49.4 v35.43,49.28
N$15  (via drill 0.35)
  Top 0.203: U1.29 27.25,29.78 27.43,29.6 27.43,28.83 26.04,27.43 v26.04,25.53 | v27.3,16 27.3,14.22 DAC4.1
  Bottom 0.203: v26.04,25.53 26.04,17.4 27.3,16.13 v27.3,16
N$16  (via drill 0.35)
  Top 0.203: U1.79 36.15,47.32 36.15,47.93 35.56,48.51 v34.67,48.51 | v27.56,56.01 27.05,56.52 USART4.1
  Bottom 0.203: v34.67,48.51 33.4,49.78 33.4,52.32 29.72,56.01 v27.56,56.01
N$17  (via drill 0.35)
  Top 0.203: U1.30 27.75,29.78 27.79,29.75 27.79,23.52 v27.81,23.49 | v36.39,14.92 37.91,14.92 SPI1.2
  Bottom 0.203: v27.81,23.49 v36.39,14.92 36.45,14.86
N$18  (via drill 0.35)
  Top 0.203: U1.31 28.35,31.42 28.35,30.81 28.45,30.71 28.45,23.75 28.57,23.62 v28.72,23.62 | v40.26,16.76 40.77,16.26 SPI1.1
  Bottom 0.203: v28.72,23.62 35.58,16.76 v40.26,16.76
N$19  (via drill 0.35)
  Top 0.203: U1.69 39.65,42.42 v41.53,42.42 | v49.28,46.99 USART1.1
  Bottom 0.203: v41.53,42.42 46.1,46.99 v49.28,46.99
N$20  (via drill 0.35)
  Top 0.203: U1.68 41.06,41.87 v41.66,41.27 | v47.75,43.56 48.01,43.56 USART1.2
  Bottom 0.203: v41.66,41.27 43.94,43.56 v47.75,43.56
N$22  (via drill 0.35)
  Top 0.203: U1.25 22.63,33.37 v22.48,33.52 | v20.57,16.13 20.57,14.1 USART2.2
  Bottom 0.203: v22.48,33.52 22.48,27.44 22.42,27.38 22.42,24.83 20.57,22.99 v20.57,16.13
N$23  (via drill 0.35)
  Top 0.203: U1.26 25.27,31.04 v25.27,29.72 | v23.37,16.38 23.37,14.1 USART2.1
  Bottom 0.203: v25.27,29.72 25.27,23.37 23.88,21.97 23.88,16.89 v23.37,16.38
N$24
  Top 0.203: R10.2 52.93,59.68 U3.5
N$25
  Top 0.203: U3.9 61.41,58.83 62,58.83 63.88,56.95 R15.2
N$26
  Top 0.203: U3.12 62.72,60.98 66.29,57.4 R16.2
NRST
  Top 0.203: U1.14 21.71,38.87 21.21,39.37 16.26,39.37 14.99,40.64 9.53,40.64 | S1.1 3.43,44.84 3.43,41.66 | 9.53,40.64 4.45,40.64 3.43,41.66 | 3.43,41.66 2.54,42.55 1.91,42.55 1.52,42.93 1.52,50.5 1.65,50.62 S1.2 3.43,50.84 3.43,52.45 | 3.43,52.45 4.32,53.34 C21.1 | 3.43,52.45 3.43,55.63 4.06,56.26 R9.1 5.33,56.31 5.33,57.02 5.59,57.28 10.16,57.28 J3.5 | J2.12 13.84,14.99 14.48,14.35 14.48,8.61 13.34,7.47 2.44,7.47 1.91,8 1.91,28.07 2.79,28.96 4.83,28.96 7.62,31.75 7.62,38.73 9.53,40.64
PC14-OSC32-IN
  Top 0.203: U1.8 22.77,41.87 21.84,42.8 21.84,44.13 Y2.2 21.91,45.78 21.34,46.36 19.05,46.36 18.8,46.61 18.8,49.53 19.3,50.04 C19.1
PC15-OSC32-OUT
  Top 0.203: U1.9 22.13,41.37 20.51,42.99 Y2.1 20.51,44.64 20.45,44.7 20.45,45.21 19.81,45.85 18.67,45.85 18.29,46.23 18.29,51.82 19.05,52.58 C20.1
PH0-OSC-IN
  Top 0.203: U1.12 21.85,39.87 20.83,40.89 19.68,40.89 16.89,43.69 16.89,49.53 | C17.1 18.92,55.37 18.16,54.61 17.27,54.61 16.89,54.23 16.89,49.53 | 16.89,49.53 16.26,50.16 15.88,50.16 15.49,50.55 Y1.2
PH1-OSC-OUT
  Top 0.203: U1.13 21.72,39.37 20.7,40.39 R8.1
SCK  (via drill 0.35)
  Top 0.203: U1.52 39.7,33.97 41.33,33.97 v41.53,34.16 | v51.69,55.63 R10.1
  Bottom 0.203: v41.53,34.16 41.53,35.31 43.81,37.59 47.62,37.59 51.69,41.66 v51.69,55.63
SCK_LLS  (via drill 0.35)
  Top 0.203: U$2.P$5 57.02,20.45 54.74,22.73 v54.74,29.21 | U3.8 61.22,41.02 58.42,38.23 v58.29,38.23
  Bottom 0.203: v58.29,38.23 55.5,35.43 52.45,35.43 52.32,35.43 50.93,34.04 50.93,31.62 53.34,29.21 v54.74,29.21
SWCLK
  Top 0.203: J2.9 12.57,10.16 11.68,9.27 10.16,9.27 9.4,10.03 9.4,14.35 9.02,14.73 8.76,14.73 8.13,15.37 8.13,18.54 8.26,18.67 9.91,18.67 10.03,18.54 J2.6 10.03,14.96 10.16,14.83 11.4,14.83 11.94,15.37 11.94,21.34 12.57,21.97 22.86,21.97 24.26,23.37 24.26,30.99 25.35,32.08 25.35,32.23 26.01,32.89 32.38,32.89 37.75,38.26 U1.76
SWDIO
  Top 0.203: U1.72 41.35,43.87 42.8,42.42 42.93,42.29 43.18,42.04 43.18,24.26 40.39,21.46 15.11,21.46 14.73,21.08 14.48,20.83 13.21,19.56 13.21,15.37 12.32,14.48 9.78,14.48 8.76,15.49 J2.4
SWO
  Top 0.203: U1.89 31.25,44.84 25.02,38.61 25.02,33.27 24.64,32.89 21.84,32.89 21.47,32.52 21.47,28.33 21.32,28.18 17.77,28.18 14.86,31.09 14.86,31.12 7.75,31.12 3.94,27.3 3.94,21.72 4.7,20.95 10.54,20.95 11.3,20.19 J2.8
USART_RX  (via drill 0.35)
  Top 0.203: U1.87 32.25,49.39 32.89,50.03 v32.89,54.61 31.88,55.63 J3.11 | v45.72,52.32 45.72,10.67 44.45,9.4 16.26,9.4 15.11,10.54 J2.13
  Bottom 0.203: v32.89,54.61 43.43,54.61 v45.72,52.32
USART_TX
  Top 0.203: U1.86 32.75,48.5 34.42,50.16 34.42,60.71 | J3.12 34.42,60.71 | 34.42,60.71 44.58,50.55 44.58,21.21 42.93,19.56 17.78,19.56 J2.14
VDDA
  Top 0.203: FB1.1 19.94,32.64 | 19.94,32.64 20.57,32.64 21.59,33.66 21.59,34.42 22.04,34.87 U1.22 | FB1.1 17.27,34.96 C13.1 | FB1.1 19.6,33.44 20.37,34.21 R7.2 | C14.A 19.94,29.51 19.94,32.64
VREF_PLUS
  Top 0.203: U1.21 23.82,35.29 C15.1 20.07,35.29 | 20.07,35.29 19.96,35.29 16.81,38.43 C16.A | R7.1 19.51,34.73 20.07,35.29

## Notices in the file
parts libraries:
SparkFun-Connectors: Licensing: Creative Commons ShareAlike 4.0 International - https://creativecommons.org/licenses/by-sa/4.0
